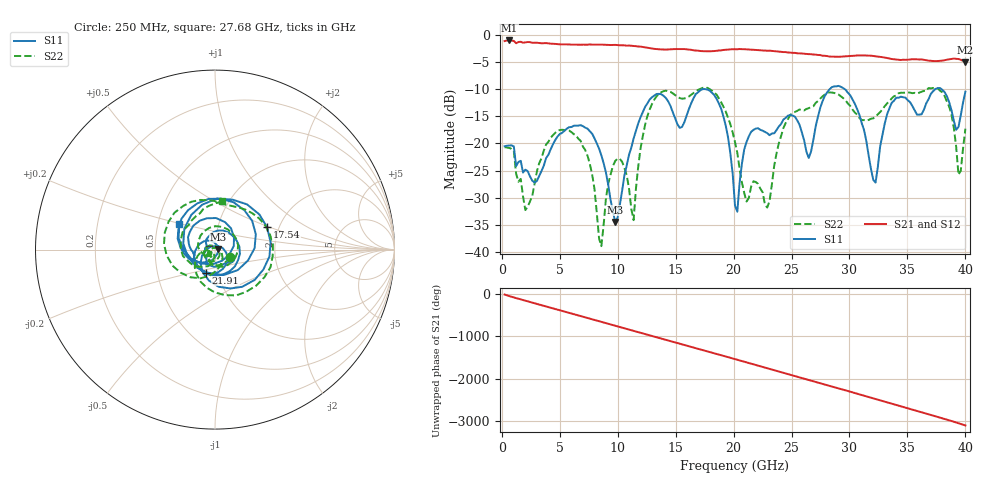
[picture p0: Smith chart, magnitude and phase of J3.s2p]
!Agilent Technologies,E8364B,MY43040528,A.07.50.67
!Agilent E8364B: A.07.50.67
!Date: Thursday, May 22, 2025 22:31:08
!Correction: S11(Full 2 Port(1,2))
!S21(Full 2 Port(1,2))
!S12(Full 2 Port(1,2))
!S22(Full 2 Port(1,2))
!S2P File: Measurements: S11, S21, S12, S22:
# Hz S  dB  R 50
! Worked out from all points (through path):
!   201 points, 250 MHz to 40 GHz, reference 50 ohm
!   highest |S21| = -1.07 dB at 647.5 MHz (marker M1); lowest = -5.1 dB at 40 GHz (marker M2)
!   group delay of S21, straight-line fit = 214 ps
!   lowest |S11| = -34.5 dB at 9.79 GHz (marker M3), VSWR 1.04, Z = 51.9 + j0.419 ohm
!   |S11| at or under -10 dB: start of sweep to 28.31 GHz; 29.57 GHz to 37.41 GHz (7.836 GHz wide, 23.4 % of centre); 37.92 GHz to end of sweep
!   |S22| runs from -38.9 to -9.8 dB; largest |S21 - S12| = 0.01
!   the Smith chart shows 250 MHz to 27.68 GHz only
!   S11 on the Smith chart (normalised r, x): 250 MHz: 1.17, -0.11; 17.54 GHz: 1.73, +0.48; 21.91 GHz: 0.88, -0.23; 27.68 GHz: 0.64, +0.19
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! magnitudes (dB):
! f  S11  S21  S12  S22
! 250 MHz  -20.5  -1.2  -1.2  -20.7
! 647.5 MHz  -20.4  -1.1  -1.0  -20.8
! 2.039 GHz  -24.8  -1.4  -1.4  -32.3
! 4.424 GHz  -20.2  -1.7  -1.7  -18.5
! 7.008 GHz  -16.8  -1.8  -1.8  -20.6
! 8.598 GHz  -22.2  -1.8  -1.8  -38.9
! 9.79 GHz  -34.5  -1.9  -1.9  -23.2
! 11.38 GHz  -19.1  -2.1  -2.1  -34.1
! 13.57 GHz  -10.9  -2.7  -2.7  -10.9
! 17.54 GHz  -10.0  -3.1  -3.0  -9.8
! 19.13 GHz  -15.1  -2.8  -2.8  -13.2
! 20.12 GHz  -31.4  -2.7  -2.7  -19.7
! 21.91 GHz  -17.3  -2.8  -2.8  -27.1
! 22.91 GHz  -18.1  -3.0  -3.0  -31.8
! 26.88 GHz  -19.4  -3.7  -3.6  -13.2
! 27.68 GHz  -12.2  -3.9  -3.8  -11.3
! 30.06 GHz  -11.1  -3.9  -3.9  -13.1
! 32.25 GHz  -27.2  -4.0  -4.0  -15.1
! 33.44 GHz  -13.6  -4.4  -4.4  -12.3
! 38.01 GHz  -10.2  -4.8  -4.8  -10.6
! 39.4 GHz  -17.0  -4.5  -4.5  -25.8
! 40 GHz  -10.5  -5.1  -5.0  -17.3
